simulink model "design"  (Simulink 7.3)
settings: Solver=ode45  StartTime=0.0  StopTime=10.0  RelTol=1e-3
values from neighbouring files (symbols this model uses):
  Kp = om^2    (= 1)    [run.m]
  Kr = 2*zt*om    (= 0.28)    [run.m]
  Q = diag([0.06, 0.005, 0.2, 0.03, 0.03, 0.03])    [run.m]
undefined symbols (not defined in the file or in its folder): Ad, Bd, Cd, Dd

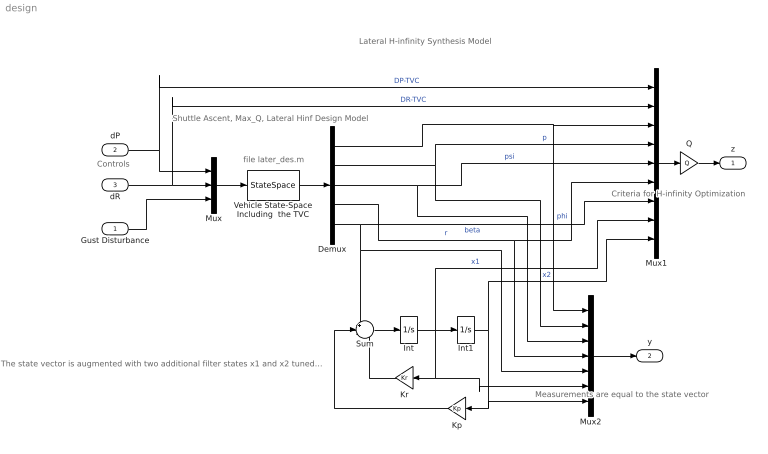
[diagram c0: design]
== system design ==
  note: The state vector is augmented with two additional filter states x1 and x2 tuned to 0.19 Hz
  note: Measurements are equal to the state vector
  note: Criteria for H-infinity Optimization
  note: Controls
  note: Shuttle Ascent, Max_Q, Lateral Hinf Design Model
  note: file later_des.m
  note: Lateral H-infinity Synthesis Model
  Gust Disturbance : Inport  OutDataType=sfix(16)  OutScaling=2^0
  dP : Inport  Port=2  OutDataType=sfix(16)  OutScaling=2^0
  dR : Inport  Port=3  OutDataType=sfix(16)  OutScaling=2^0
  Demux : Demux  Outputs=5
  Int : Integrator
  Int1 : Integrator
  Kp : Gain  Gain=Kp  ParameterDataType=sfix(16)  ParameterScaling=2^0  OutDataType=sfix(16)  OutScaling=2^0
  Kr : Gain  Gain=Kr  ParameterDataType=sfix(16)  ParameterScaling=2^0  OutDataType=sfix(16)  OutScaling=2^0
  Mux : Mux  Inputs=3
  Mux1 : Mux  Inputs=9
  Mux2 : Mux  Inputs=7
  Q : Gain  Gain=Q  Multiplication=Matrix(K*u)  ParameterDataType=sfix(16)  ParameterScaling=2^0  OutDataType=sfix(16)  OutScaling=2^0
  Sum : Sum  Inputs=+--  OutDataType=sfix(16)  OutScaling=2^0
  Vehicle State-Space Including  the TVC : StateSpace  A=Ad  B=Bd  C=Cd  D=Dd
  z : Outport  OutDataType=sfix(16)  OutScaling=2^0
  y : Outport  Port=2  OutDataType=sfix(16)  OutScaling=2^0
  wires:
  Vehicle State-Space Including  the TVC/1 -> Demux/1
  Mux/1 -> Vehicle State-Space Including  the TVC/1
  Demux/1 -> Mux2/1, Mux1/3  "phi"
  dP/1 -> Mux/1, Mux1/1  "DP-TVC"
  dR/1 -> Mux/2, Mux1/2  "DR-TVC"
  Demux/2 -> Mux2/2, Mux1/4  "p"
  Demux/3 -> Mux2/3, Mux1/5  "psi"
  Demux/4 -> Mux2/4, Mux1/6  "r"
  Demux/5 -> Sum/1, Mux2/5, Mux1/7  "beta"
  Int/1 -> Int1/1, Kr/1, Mux2/6, Mux1/8  "x1"
  Sum/1 -> Int/1
  Int1/1 -> Kp/1, Mux2/7, Mux1/9  "x2"
  Kr/1 -> Sum/3
  Kp/1 -> Sum/2
  Gust Disturbance/1 -> Mux/3
  Mux1/1 -> Q/1
  Mux2/1 -> y/1
  Q/1 -> z/1
